(* Logix 5000 AddOnInstructionDefinition export AOI_MGB; software revision 20.03 *)

TYPE MGB_Safety_Tags_Type :   // These are the safety Input and Output Tags of the MGB -
STRUCT
   InputData : MGB_Safety_In_Data_Type;   // Safety Input Data which will be recived from the MAB
   OutputData : MGB_Safety_Out_Data_Type;   // Safety Output Data which will be send to the MAB
END_STRUCT
END_TYPE

TYPE MGB_Std_Out_Data :   // These are the standard output Tags of the MGB
STRUCT
   H90 : BOOL;   // Operator Indicator - controls illumination of the operator 1 = illumination is turned ON 0 = illumination is turned OFF
   H91 : BOOL;   // Operator Indicator - controls illumination of the operator 1 = illumination is turned ON 0 = illumination is turned OFF
   H92 : BOOL;   // Operator Indicator - controls illumination of the operator 1 = illumination is turned ON 0 = illumination is turned OFF
   H93 : BOOL;   // Operator Indicator - controls illumination of the operator 1 = illumination is turned ON 0 = illumination is turned OFF
   H94 : BOOL;   // Operator Indicator - controls illumination of the operator 1 = illumination is turned ON 0 = illumination is turned OFF
   H95 : BOOL;   // Operator Indicator - controls illumination of the operator 1 = illumination is turned ON 0 = illumination is turned OFF
   H1 : BOOL;   // Operator Indicator - controls illumination of the operator 1 = illumination is turned ON 0 = illumination is turned OFF
   H2 : BOOL;   // Operator Indicator - controls illumination of the operator 1 = illumination is turned ON 0 = illumination is turned OFF
   H3 : BOOL;   // Operator Indicator - controls illumination of the operator 1 = illumination is turned ON 0 = illumination is turned OFF
   H4 : BOOL;   // Operator Indicator - controls illumination of the operator 1 = illumination is turned ON 0 = illumination is turned OFF
   Q_G : BOOL;   // General Fault Acknowledgement - resets the bus module 1=Reset of bus module 0=normal operation of device
   Q_PF : BOOL;   // Lock Module Fault Acknowledgement - resets the lock module 1=Reset of locking module 0=normal operation of device
END_STRUCT
END_TYPE

TYPE MGB_Safety_Out_Data_Type :   // These are the safety output Tags of the MGB
STRUCT
   FO_CL : BOOL;   // Lock Command - control for switching the guard locking on and off 0 = Guardlocking is locked 1 = Guardlocking is unlocked
END_STRUCT
END_TYPE

TYPE MGB_Std_In_Data_Type :   // These are the standard input Tags of the MGB
STRUCT
   RunMode : BOOL;   // Run Mode - Indicates the operating mode of the access box 0 = while restarting 1 = Run Mode after successful restarting of bus module
   ConnectionFaulted : BOOL;   // Connection Faulted - Indicates the state of the communication connection between the access box and the controller. 0 = Connection of output data 1 = Connection of output data Faulted
   DiagnosticActive : BOOL;   // Diagnostic Active - Indicates whether the access box is faulted. 0 = No Fault 1 = Fault
   DiagnosticSequenceCount : SINT;   // Diagnostic Sequence Count - Displays the total accumulated diagnostic counts. Values range from 0…255.
   S90_1 : BOOL;   // Operator Position S90 1 = Pressed (push button) or right position (selector switch) 0 = Released (push button) or 2-position selector switch in middle position or 3-position selector switch
   S91_1 : BOOL;   // Operator Position S91 1 = Pressed (push button) or right position (selector switch) 0 = Released (push button) or 2-position selector switch in middle position or 3-position selector switch
   S92_1 : BOOL;   // Operator Position 92 1 = Pressed (push button) or right position (selector switch) 0 = Released (push button) or 2-position selector switch in middle position or 3-position selector switch
   S93_1 : BOOL;   // Operator Position 93 1 = Pressed (push button) or right position (selector switch) 0 = Released (push button) or 2-position selector switch in middle position or 3-position selector switch
   S94_1 : BOOL;   // Operator Position 94 1 = Pressed (push button) or right position (selector switch) 0 = Released (push button) or 2-position selector switch in middle position or 3-position selector switch
   S95_1 : BOOL;   // Operator Position 95 1 = Pressed (push button) or right position (selector switch) 0 = Released (push button) or 2-position selector switch in middle position or 3-position selector switch
   S1_1 : BOOL;   // Operator Position S1 1 = Pressed (push button) or right position (selector switch) 0 = Released (push button) or 2-position selector switch in middle position or 3-position selector switch
   S2_1 : BOOL;   // Operator Position S2 1 = Pressed (push button) or right position (selector switch) 0 = Released (push button) or 2-position selector switch in middle position or 3-position selector switch
   S3_1 : BOOL;   // Operator Position S3 1 = Pressed (push button) or right position (selector switch) 0 = Released (push button) or 2-position selector switch in middle position or 3-position selector switch
   S4_1 : BOOL;   // Operator Position S4 1 = Pressed (push button) or right position (selector switch) 0 = Released (push button) or 2-position selector switch in middle position or 3-position selector switch
   S90_2 : BOOL;   // Operator Position S90 1 = left position (3-position selector switch) 0 = released push button or 2 position selector switch in right or middle position or 3 position selector switch in middle position
   S91_2 : BOOL;   // Operator Position S91 1 = left position (3-position selector switch) 0 = released push button or 2 position selector switch in right or middle position or 3 position selector switch in middle position
   S92_2 : BOOL;   // Operator Position 92 1 = left position (3-position selector switch) 0 = released push button or 2 position selector switch in right or middle position or 3 position selector switch in middle position
   S93_2 : BOOL;   // Operator Position 93 1 = left position (3-position selector switch) 0 = released push button or 2 position selector switch in right or middle position or 3 position selector switch in middle position
   S94_2 : BOOL;   // Operator Position 94 1 = left position (3-position selector switch) 0 = released push button or 2 position selector switch in right or middle position or 3 position selector switch in middle position
   S95_2 : BOOL;   // Operator Position 95 1 = left position (3-position selector switch) 0 = released push button or 2 position selector switch in right or middle position or 3 position selector switch in middle position
   S1_2 : BOOL;   // Operator Position S1 1 = left position (3-position selector switch) 0 = released push button or 2 position selector switch in right or middle position or 3 position selector switch in middle position
   S2_2 : BOOL;   // Operator Position S2 1 = left position (3-position selector switch) 0 = released push button or 2 position selector switch in right or middle position or 3 position selector switch in middle position
   S3_2 : BOOL;   // Operator Position S3 1 = left position (3-position selector switch) 0 = released push button or 2 position selector switch in right or middle position or 3 position selector switch in middle position
   S4_2 : BOOL;   // Operator Position S4 1 = left position (3-position selector switch) 0 = released push button or 2 position selector switch in right or middle position or 3 position selector switch in middle position
   D_PF : BOOL;   // Plausability Fault - indicates a signal sequence error (lock module error)
   D_ES : BOOL;   // Estop Fault - indicates an E-stop specific fault
   D_EN : BOOL;   // Enabling Switch Fault - indicates an Enabling Switch specific fault
   D_MS : BOOL;   // Safe Mode Selector Switch Fault - indicates a Mode Selector Switch specific fault
   D_OL : BOOL;   // Lock Command Fault - indicates a fault in the Lock Command
   D_LT : BOOL;   // Cycle Count - indicates when the device has reached more than 1,000,000 switching cycles 0 = < 1,000,000 swtiching cycles of the solenoid 1 = > 1,000,000 switching cylcles of the solenoid
   FaultCode1 : SINT;   // Fault Code1 - indicates the specific diagnostic message of the access box
   FaultCode2 : SINT;   // Fault Code2 - indicates the specific diagnostic message of the access box
   FaultCode : INT;   // Fault Code - indicates the specific diagnostic message of the access box
END_STRUCT
END_TYPE

TYPE MGB_Safety_In_Data_Type :   // These are the safety input Tags of the MGB
STRUCT
   FI_ES : BOOL;   // E-stop Button Status 1 = Contacts Closed (E-stop not pressed) 0 = Contacts Open (E-stop pressed)
   FI_EN : BOOL;   // Enabling Switch Status 1 = Switch Enabled 0 = Released
   FI_MS0 : BOOL;   // Operating Mode Selector Switch 1 = Selector Switch in position 1 0 = Selector switch is not in position 1
   FI_MS1 : BOOL;   // Operating Mode Selector Switch 1 = Selector Switch in position 2 0 = Selector switch is not in position 2
   FI_MS2 : BOOL;   // Operating Mode Selector Switch 1 = Selector Switch in position 3 0 = Selector switch is not in position 3
   FI_D : BOOL;   // Door Status - position of the guard door 0 = guard door is OPEN 1 = guard door is CLOSED
   FI_B : BOOL;   // Bolt Status - position of the bolt actuator 0 = bolt is retracted 1 = bolt is extended
   FI_L : BOOL;   // Solenoid Status - position of the solenoid locking arm 0 = locking arm is in unlocked position 1 = locking arm is in locked position
   FI_SK : BOOL;   // Interlock Status 0 = bolt retracted and/or door OPEN 1 = door is CLOSED and bolt is extended
   FI_UK : BOOL;   // Guard Lock Status 0 = door is OPEN, or door is CLOSED with bolt retracted, or door is CLOSED with bolt extended and unlocked 1 = door is CLOSED, bolt is extended, and bolt is locked
END_STRUCT
END_TYPE

ADD_ON_INSTRUCTION AOI_MGB   (* revision 1.0 Basic Version, vendor EUCHNER GmbH + Co. KG, safety *)
// Defines datastructure for all MGB-Ethernet/IP. Copying data from MGB into different UDTs describing MGB like in manual..
// Usage described in application AP000224 and using application AP000223
// Revision note:
// Initial version of this AOI
// Help:
// Please use application AP000223 and application AP000224 for understanding usage of this AOI. Download is available on EUCHNER homepage www.euchner.com
VAR_OUTPUT
   RunMode : BOOL; {visible}
   ConnectionFaulted : BOOL; {visible}
   FaultCode : INT; {access Read Only, visible}
END_VAR
VAR_IN_OUT
   MGB_Device_Input_Data : AB:ETHERNET_SAFETYMODULE_16Bytes:I:0; {required}
   MGB_Device_Output_Data : AB:ETHERNET_SAFETYMODULE_4Bytes:O:0; {required}
   MGB_Safety_Tags : MGB_Safety_Tags_Type; {required}
   MGB_Standard_Input_Tags : MGB_Std_In_Data_Type; {required}
   MGB_Standard_Output_Tags : MGB_Std_Out_Data; {required}
END_VAR

ROUTINE Logic   (* ladder *)
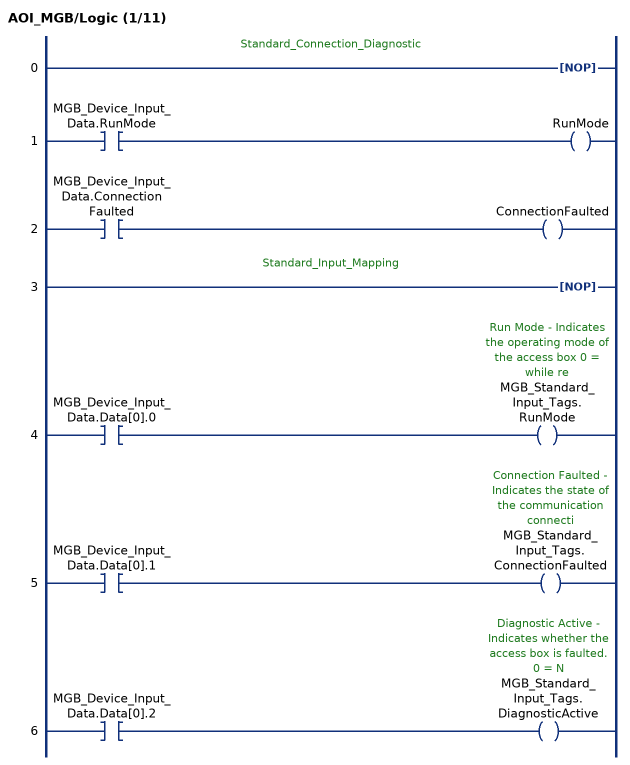
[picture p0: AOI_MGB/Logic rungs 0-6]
   // Standard_Connection_Diagnostic
   0: NOP();
   1: XIC(MGB_Device_Input_Data.RunMode)OTE(RunMode);
   2: XIC(MGB_Device_Input_Data.ConnectionFaulted)OTE(ConnectionFaulted);
   // Standard_Input_Mapping
   3: NOP();
   4: XIC(MGB_Device_Input_Data.Data[0].0)OTE(MGB_Standard_Input_Tags.RunMode);
   5: XIC(MGB_Device_Input_Data.Data[0].1)OTE(MGB_Standard_Input_Tags.ConnectionFaulted);
   6: XIC(MGB_Device_Input_Data.Data[0].2)OTE(MGB_Standard_Input_Tags.DiagnosticActive);
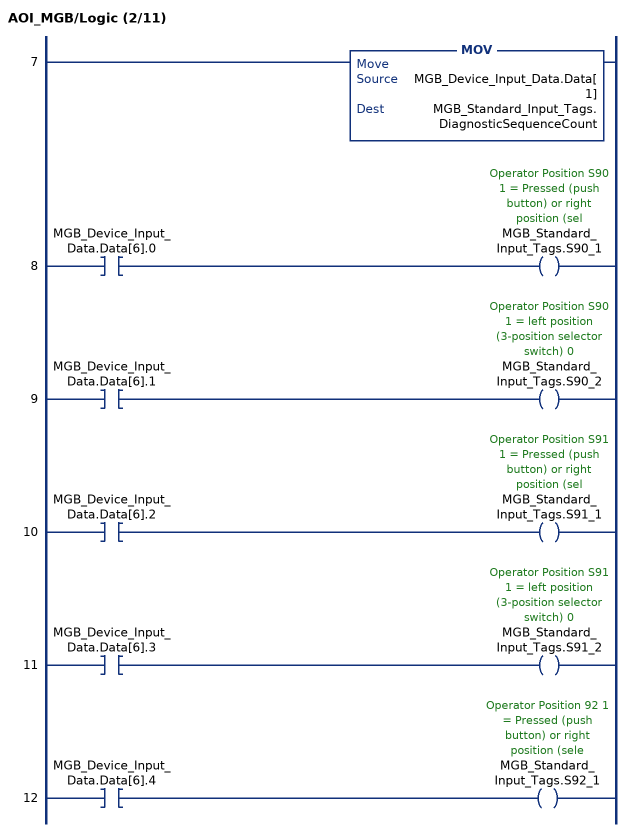
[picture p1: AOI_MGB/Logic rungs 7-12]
   7: MOV(MGB_Device_Input_Data.Data[1],MGB_Standard_Input_Tags.DiagnosticSequenceCount);
   8: XIC(MGB_Device_Input_Data.Data[6].0)OTE(MGB_Standard_Input_Tags.S90_1);
   9: XIC(MGB_Device_Input_Data.Data[6].1)OTE(MGB_Standard_Input_Tags.S90_2);
   10: XIC(MGB_Device_Input_Data.Data[6].2)OTE(MGB_Standard_Input_Tags.S91_1);
   11: XIC(MGB_Device_Input_Data.Data[6].3)OTE(MGB_Standard_Input_Tags.S91_2);
   12: XIC(MGB_Device_Input_Data.Data[6].4)OTE(MGB_Standard_Input_Tags.S92_1);
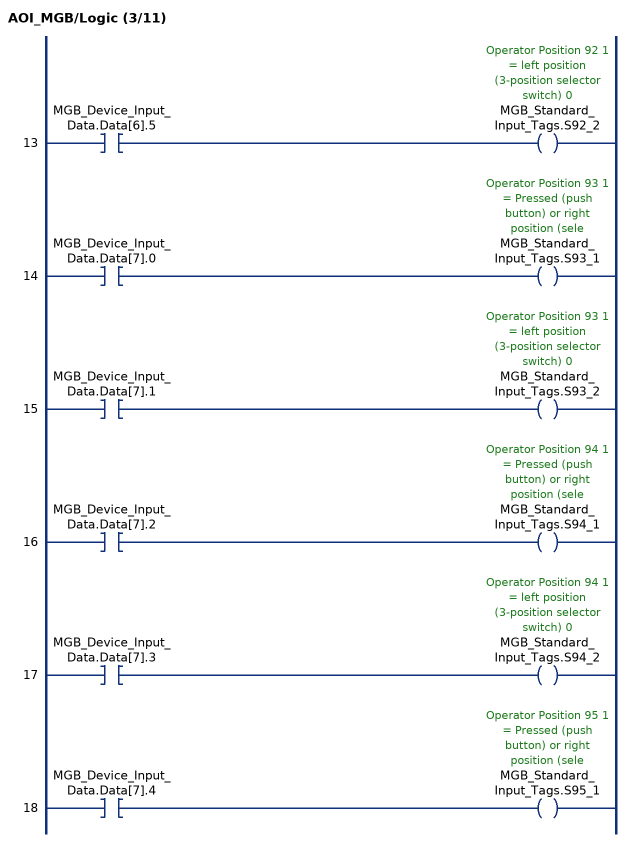
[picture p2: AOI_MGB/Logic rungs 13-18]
   13: XIC(MGB_Device_Input_Data.Data[6].5)OTE(MGB_Standard_Input_Tags.S92_2);
   14: XIC(MGB_Device_Input_Data.Data[7].0)OTE(MGB_Standard_Input_Tags.S93_1);
   15: XIC(MGB_Device_Input_Data.Data[7].1)OTE(MGB_Standard_Input_Tags.S93_2);
   16: XIC(MGB_Device_Input_Data.Data[7].2)OTE(MGB_Standard_Input_Tags.S94_1);
   17: XIC(MGB_Device_Input_Data.Data[7].3)OTE(MGB_Standard_Input_Tags.S94_2);
   18: XIC(MGB_Device_Input_Data.Data[7].4)OTE(MGB_Standard_Input_Tags.S95_1);
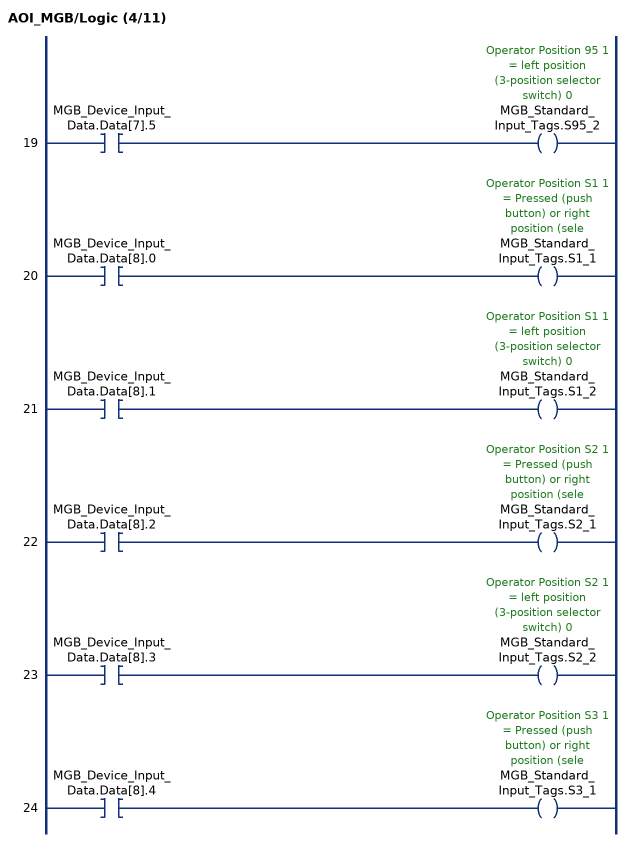
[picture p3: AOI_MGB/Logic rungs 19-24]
   19: XIC(MGB_Device_Input_Data.Data[7].5)OTE(MGB_Standard_Input_Tags.S95_2);
   20: XIC(MGB_Device_Input_Data.Data[8].0)OTE(MGB_Standard_Input_Tags.S1_1);
   21: XIC(MGB_Device_Input_Data.Data[8].1)OTE(MGB_Standard_Input_Tags.S1_2);
   22: XIC(MGB_Device_Input_Data.Data[8].2)OTE(MGB_Standard_Input_Tags.S2_1);
   23: XIC(MGB_Device_Input_Data.Data[8].3)OTE(MGB_Standard_Input_Tags.S2_2);
   24: XIC(MGB_Device_Input_Data.Data[8].4)OTE(MGB_Standard_Input_Tags.S3_1);
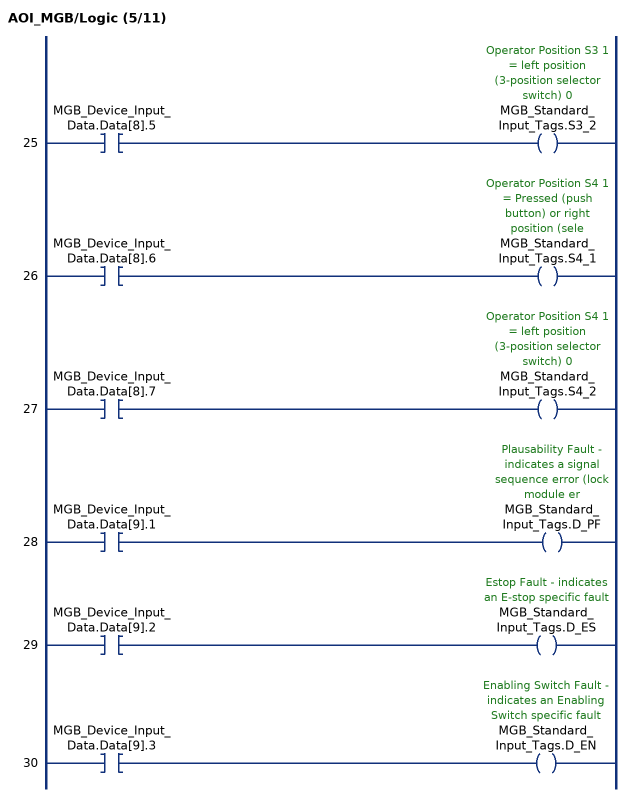
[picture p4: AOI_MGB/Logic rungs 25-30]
   25: XIC(MGB_Device_Input_Data.Data[8].5)OTE(MGB_Standard_Input_Tags.S3_2);
   26: XIC(MGB_Device_Input_Data.Data[8].6)OTE(MGB_Standard_Input_Tags.S4_1);
   27: XIC(MGB_Device_Input_Data.Data[8].7)OTE(MGB_Standard_Input_Tags.S4_2);
   28: XIC(MGB_Device_Input_Data.Data[9].1)OTE(MGB_Standard_Input_Tags.D_PF);
   29: XIC(MGB_Device_Input_Data.Data[9].2)OTE(MGB_Standard_Input_Tags.D_ES);
   30: XIC(MGB_Device_Input_Data.Data[9].3)OTE(MGB_Standard_Input_Tags.D_EN);
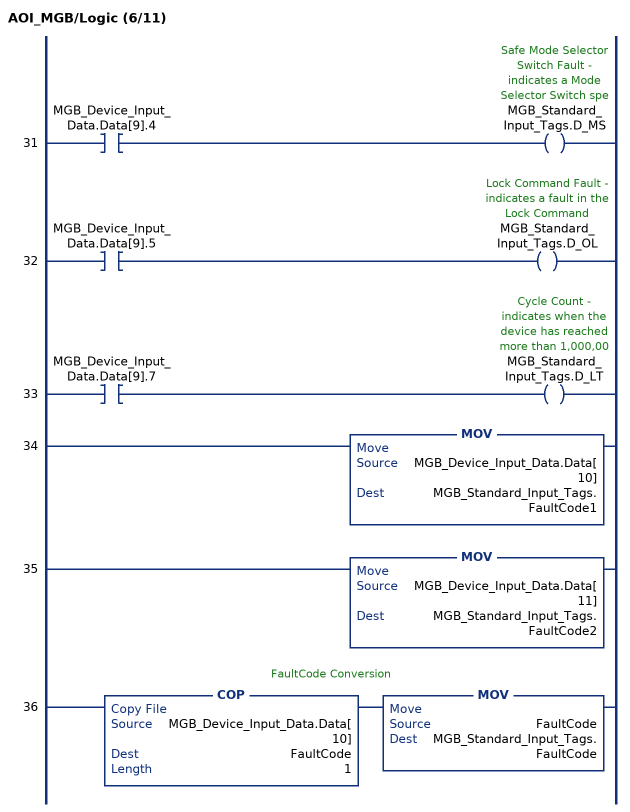
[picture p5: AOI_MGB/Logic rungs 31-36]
   31: XIC(MGB_Device_Input_Data.Data[9].4)OTE(MGB_Standard_Input_Tags.D_MS);
   32: XIC(MGB_Device_Input_Data.Data[9].5)OTE(MGB_Standard_Input_Tags.D_OL);
   33: XIC(MGB_Device_Input_Data.Data[9].7)OTE(MGB_Standard_Input_Tags.D_LT);
   34: MOV(MGB_Device_Input_Data.Data[10],MGB_Standard_Input_Tags.FaultCode1);
   35: MOV(MGB_Device_Input_Data.Data[11],MGB_Standard_Input_Tags.FaultCode2);
   // FaultCode Conversion
   36: COP(MGB_Device_Input_Data.Data[10],FaultCode,1)MOV(FaultCode,MGB_Standard_Input_Tags.FaultCode);
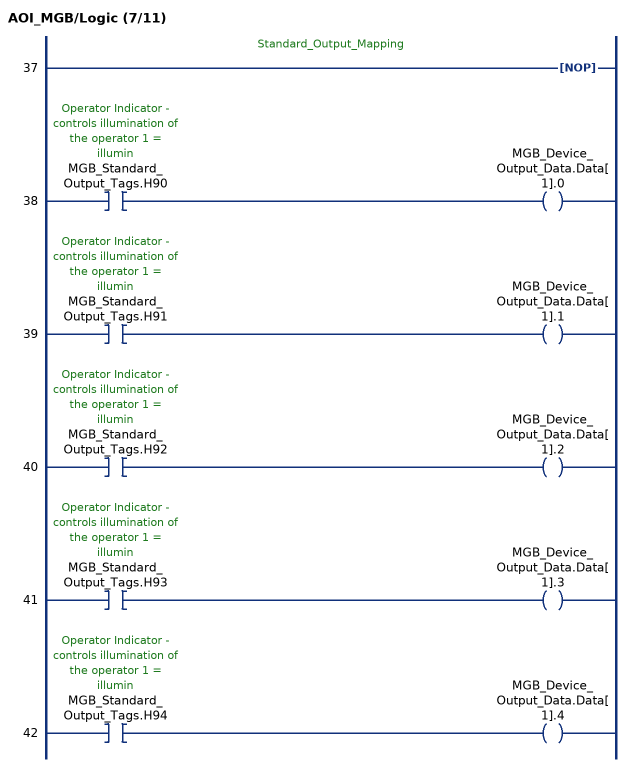
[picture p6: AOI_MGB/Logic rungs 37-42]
   // Standard_Output_Mapping
   37: NOP();
   38: XIC(MGB_Standard_Output_Tags.H90)OTE(MGB_Device_Output_Data.Data[1].0);
   39: XIC(MGB_Standard_Output_Tags.H91)OTE(MGB_Device_Output_Data.Data[1].1);
   40: XIC(MGB_Standard_Output_Tags.H92)OTE(MGB_Device_Output_Data.Data[1].2);
   41: XIC(MGB_Standard_Output_Tags.H93)OTE(MGB_Device_Output_Data.Data[1].3);
   42: XIC(MGB_Standard_Output_Tags.H94)OTE(MGB_Device_Output_Data.Data[1].4);
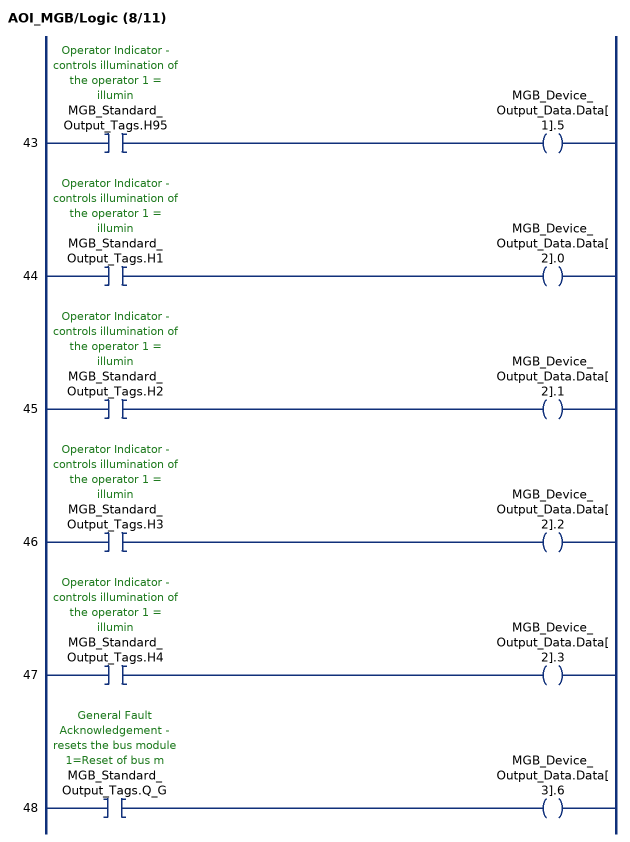
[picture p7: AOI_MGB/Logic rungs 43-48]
   43: XIC(MGB_Standard_Output_Tags.H95)OTE(MGB_Device_Output_Data.Data[1].5);
   44: XIC(MGB_Standard_Output_Tags.H1)OTE(MGB_Device_Output_Data.Data[2].0);
   45: XIC(MGB_Standard_Output_Tags.H2)OTE(MGB_Device_Output_Data.Data[2].1);
   46: XIC(MGB_Standard_Output_Tags.H3)OTE(MGB_Device_Output_Data.Data[2].2);
   47: XIC(MGB_Standard_Output_Tags.H4)OTE(MGB_Device_Output_Data.Data[2].3);
   48: XIC(MGB_Standard_Output_Tags.Q_G)OTE(MGB_Device_Output_Data.Data[3].6);
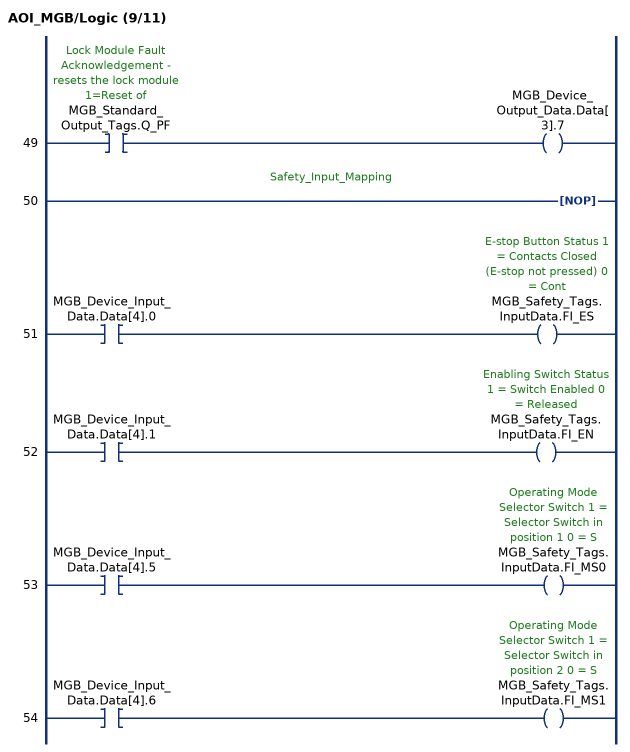
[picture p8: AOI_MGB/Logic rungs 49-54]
   49: XIC(MGB_Standard_Output_Tags.Q_PF)OTE(MGB_Device_Output_Data.Data[3].7);
   // Safety_Input_Mapping
   50: NOP();
   51: XIC(MGB_Device_Input_Data.Data[4].0)OTE(MGB_Safety_Tags.InputData.FI_ES);
   52: XIC(MGB_Device_Input_Data.Data[4].1)OTE(MGB_Safety_Tags.InputData.FI_EN);
   53: XIC(MGB_Device_Input_Data.Data[4].5)OTE(MGB_Safety_Tags.InputData.FI_MS0);
   54: XIC(MGB_Device_Input_Data.Data[4].6)OTE(MGB_Safety_Tags.InputData.FI_MS1);
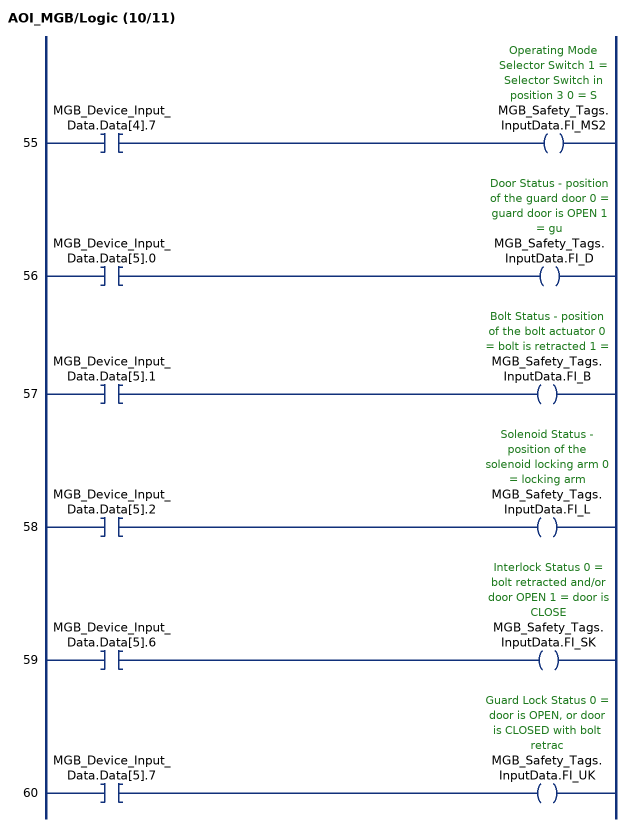
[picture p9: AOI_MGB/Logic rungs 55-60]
   55: XIC(MGB_Device_Input_Data.Data[4].7)OTE(MGB_Safety_Tags.InputData.FI_MS2);
   56: XIC(MGB_Device_Input_Data.Data[5].0)OTE(MGB_Safety_Tags.InputData.FI_D);
   57: XIC(MGB_Device_Input_Data.Data[5].1)OTE(MGB_Safety_Tags.InputData.FI_B);
   58: XIC(MGB_Device_Input_Data.Data[5].2)OTE(MGB_Safety_Tags.InputData.FI_L);
   59: XIC(MGB_Device_Input_Data.Data[5].6)OTE(MGB_Safety_Tags.InputData.FI_SK);
   60: XIC(MGB_Device_Input_Data.Data[5].7)OTE(MGB_Safety_Tags.InputData.FI_UK);
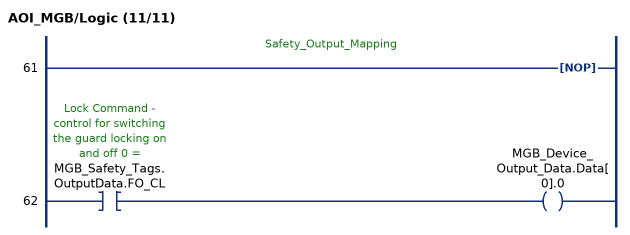
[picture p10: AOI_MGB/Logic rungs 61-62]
   // Safety_Output_Mapping
   61: NOP();
   62: XIC(MGB_Safety_Tags.OutputData.FO_CL)OTE(MGB_Device_Output_Data.Data[0].0);
END_ROUTINE
END_ADD_ON_INSTRUCTION
